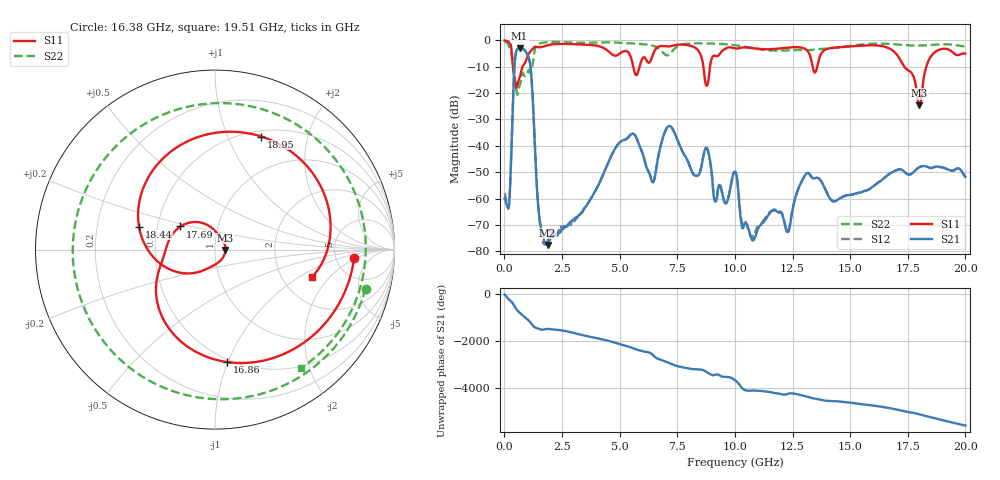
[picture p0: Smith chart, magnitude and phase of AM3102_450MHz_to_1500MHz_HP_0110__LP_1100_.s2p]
!Agilent Technologies,E8364B,MY43040894,A.07.50.67
!Agilent E8364B: A.07.50.67
!Date: Thursday, January 11, 2018 05:49:28
!Correction: S11(Full 2 Port(1,2))
!S21(Full 2 Port(1,2))
!S12(Full 2 Port(1,2))
!S22(Full 2 Port(1,2))
!S2P File: Measurements: S11, S21, S12, S22:
# Hz S  dB  R 50
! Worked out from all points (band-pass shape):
!   1601 points, 10 MHz to 20 GHz, reference 50 ohm
!   highest |S21| = -3.05 dB at 659.7 MHz (marker M1); lowest = -77.6 dB at 1.872 GHz (marker M2)
!   |S21| within 3 dB of the highest: 475.2 MHz to 1.027 GHz (552.1 MHz wide, 73.5 % of centre)
!   lowest |S11| = -24.7 dB at 18 GHz (marker M3), VSWR 1.12, Z = 56.2 - j0.212 ohm
!   |S11| at or under -10 dB: 371.1 MHz to 784.3 MHz (413.1 MHz wide, 71.5 % of centre); 8.635 GHz to 8.921 GHz (285.1 MHz wide, 3.25 % of centre); 17.35 GHz to 18.3 GHz (951.8 MHz wide, 5.34 % of centre)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
!   |S22| runs from -20.6 to -0.5 dB; largest |S21 - S12| = 0.0026
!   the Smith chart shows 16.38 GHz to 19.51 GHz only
!   S11 on the Smith chart (normalised r, x): 16.38 GHz: 7.52, -1.80; 16.86 GHz: 0.48, -0.99; 17.69 GHz: 0.66, +0.18; 18.44 GHz: 0.39, +0.13; 18.95 GHz: 0.57, +1.33; 19.51 GHz: 2.92, -1.31
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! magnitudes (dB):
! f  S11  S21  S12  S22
! 10 MHz  -0.1  -59.9  -58.0  -0.5
! 197.4 MHz  -0.7  -62.7  -62.7  -2.3
! 459.8 MHz  -15.9  -7.3  -7.3  -14.5
! 659.7 MHz  -14.2  -3.0  -3.0  -17.3
! 1.097 GHz  -4.6  -8.1  -8.1  -12.3
! 1.509 GHz  -2.7  -66.5  -67.0  -1.3
! 1.872 GHz  -1.9  -77.6  -76.0  -0.7
! 3.346 GHz  -1.6  -65.2  -65.6  -0.9
! 5.057 GHz  -4.7  -38.3  -38.3  -0.9
! 6.682 GHz  -2.4  -43.8  -43.8  -3.0
! 10.01 GHz  -3.1  -49.8  -49.8  -1.9
! 10.79 GHz  -3.0  -75.5  -74.2  -3.0
! 13.34 GHz  -8.6  -52.0  -51.9  -3.6
! 16.38 GHz  -2.2  -52.9  -52.9  -1.2
! 16.68 GHz  -3.0  -50.8  -50.8  -1.3
! 16.86 GHz  -4.0  -49.8  -49.7  -1.5
! 17.69 GHz  -12.7  -50.5  -50.4  -2.0
! 18 GHz  -24.7  -48.1  -48.1  -2.0
! 18.44 GHz  -7.1  -48.3  -48.3  -1.8
! 18.95 GHz  -3.3  -48.1  -48.1  -1.5
! 19.51 GHz  -5.0  -49.3  -49.2  -1.8
! 20 GHz  -5.0  -51.7  -52.0  -2.4
